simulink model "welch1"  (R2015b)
settings: Solver=ode45  StartTime=0.0  StopTime=10  RelTol=1e-3
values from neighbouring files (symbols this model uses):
  fs = 4000    [abtast_rate_1.m]    (also in ad_test_12.m = ',     num2str(fs),'; ad_test_2.m = ',     num2str(fs),'; ad_test_3.m = ',     num2str(fs),'; DA_wandler_spektr_1.m = 100)
  nfft = 2^p2    [DA_wandler_spektr_1.m]    (also in DA_wandler_spektr_2.m; PSD_korrelation_1.m = 2^(nextpow2(2*lag_max)); welch_1.m = 256; zero_padd1.m = ',num2str(nfft),')
  pw = sum(hanning(N).^2)/N    [leakage_2.m]    (also in leakage_3.m; leakage_4.m; welch_1.m = sum(hamming(nfft).^2)/nfft; zero_padd2.m = sum(hamming(N).^2)/N)
  Ts = 1/fs    (= 0.00025)    [abtast_rate_1.m]    (also in ad_test_12.m = 0.0009765625; ad_test_2.m = 0.00048828125; ad_test_3.m = 0.00048828125; DA_wandler_spektr_1.m = 0.01)
undefined symbols (not defined in the file or in its folder): fdesignblkfcn, Fs, gcbh, get
libraries: dspspect3 x2, dspstat3 x2, dspsnks4 x2, dspsigops x1

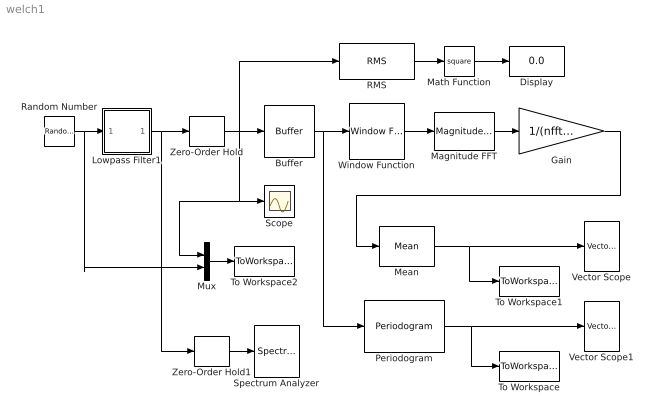
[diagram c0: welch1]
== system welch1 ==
  Buffer : Buffer  N=nfft  V=nfft/2  TreatMby1Signals=One channel
  Display : Display
  Gain : Gain  Gain=1/(nfft*pw*fs)
  Lowpass Filter1 : Subsystem  DialogController=fdesignblkfcn  InitFcn=fdesignblkfcn(gcbh, {'InitFcn'});
  Magnitude FFT : dspspect3/Magnitude FFT  mag_or_magsq=Magnitude squared  FFTImplementation=Auto  fftLenInherit=off  fftsize=nfft  WrapInput=off
  Math Function : Math  Operator=square
  Mean : dspstat3/Mean  run=on  reset_popup=None  directionMode=Each column  dimension=1  roiEnable=off  roiType=Rectangles  roiPortion=Entire ROI  roiOutput=Individual statistics for each ROI  roiFlag=off  outputDataTypeStr=Inherit: Same as accumulator  outputLastDataTypeStr=Inherit: Same as accumulator  outputMin=[]  outputMax=[]  roundingMode=Floor  overflowMode=off
  Mux : Mux  Inputs=2
  Periodogram : dspspect3/Periodogram  measurement=Power spectral density  wintype=Hamming  Rs=50  beta=5  winsamp=Symmetric  FFTImplementation=Auto  inheritFFT=off  fftsize=nfft  navg=50  inheritTs=on  Ts=1
  RMS : dspstat3/RMS  run=on  reset_popup=None  directionMode=Each column  dimension=1
  Random Number : RandomNumber  SampleTime=Ts
  Scope : Scope
  Spectrum Analyzer : SpectrumAnalyzer
  To Workspace : ToWorkspace  VariableName=Sxxw  SaveFormat=Structure  SampleTime=-1
  To Workspace1 : ToWorkspace  VariableName=Sxx  SaveFormat=Structure  SampleTime=-1
  To Workspace2 : ToWorkspace  VariableName=x  SaveFormat=Structure With Time  SampleTime=-1
  Vector Scope : dspsnks4/Vector Scope  ScopeProperties=on  Domain=Frequency  HorizSpan=1  DisplayProperties=off  AxisGrid=on  Memory=off  FrameNumber=on  AxisLegend=off  AxisZoom=off  OpenScopeAtSimStart=on  OpenScopeImmediately=off  FigPos=get(0,'defaultfigureposition')  AxisProperties=off  XUnits=Hertz  XRange=[-Fs/2...Fs/2]  InheritXIncr=off  XIncr=Ts  XLabel=Time  XLimit=Auto  XMin=0  XMax=1000  XStart=0  YUnits=dB  YLabel=Amplitude  LineProperties=off  XAxisParamsVer=6.9
  Vector Scope1 : dspsnks4/Vector Scope  ScopeProperties=on  Domain=Frequency  HorizSpan=1  DisplayProperties=off  AxisGrid=on  Memory=off  FrameNumber=on  AxisLegend=off  AxisZoom=off  OpenScopeAtSimStart=on  OpenScopeImmediately=off  FigPos=[384 509 560 420]  AxisProperties=off  XUnits=Hertz  XRange=[-Fs/2...Fs/2]  InheritXIncr=off  XIncr=Ts  XLabel=Time  XLimit=Auto  XMin=0  XMax=1000  XStart=0  YUnits=dB  YLabel=Amplitude  LineProperties=off  XAxisParamsVer=6.9
  Window Function : dspsigops/Window Function  winmode=Apply window to input  wintype=Hamming  sampmode=Continuous  samptime=1  N=64  Rs=50  beta=10  winsamp=Symmetric  UserWindow=hamming  OptParams=off  UserParams={'symmetric'}  dataType=double  isSigned=on  wordLen=16  udDataType=sfix(16)  fracBitsMode=Best precision  numFracBits=15  roundingMode=Floor  overflowMode=off  numSidelobes=4  sidelobeLevel=-30
  Zero-Order Hold : ZeroOrderHold  SampleTime=Ts
  Zero-Order Hold1 : ZeroOrderHold  SampleTime=Ts
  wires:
  Random Number/1 -> Mux/2, Lowpass Filter1/1(In)
  Zero-Order Hold/1 -> RMS/1, Scope/1, Mux/1, Buffer/1
  Window Function/1 -> Magnitude FFT/1
  Magnitude FFT/1 -> Gain/1
  RMS/1 -> Math Function/1
  Buffer/1 -> Periodogram/1, Window Function/1
  Gain/1 -> Mean/1
  Zero-Order Hold1/1 -> Spectrum Analyzer/1
  Mean/1 -> To Workspace1/1, Vector Scope/1
  Periodogram/1 -> To Workspace/1, Vector Scope1/1
  Math Function/1 -> Display/1
  Lowpass Filter1/1(Out) -> Zero-Order Hold1/1, Zero-Order Hold/1
  Mux/1 -> To Workspace2/1

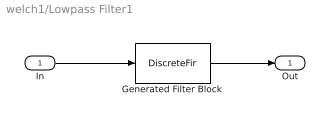
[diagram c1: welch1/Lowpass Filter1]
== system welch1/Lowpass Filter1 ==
  In : Inport
  Generated Filter Block : DiscreteFir  Tag=BlockMethodSubSystem  Coefficients=[-0.00184968043930577083 -0.00310320049717134876 -0.00190078685653537411 0.0029665306410957739 0.00894658665127252145 0.0113172677007358138 0.00781130151730347055 0.00147698486076727926 -0.00208242916168058321 -0.00056383609450246625 0.00275307531797207555 0.00315932284860923757 0.000157843099805887906 -0.00231006391432280389 -0.00120556490852751072 0.00167549984802898297 0.00227248524735140572 -0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
  Out : Outport
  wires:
  Generated Filter Block/1 -> Out/1
  In/1 -> Generated Filter Block/1
